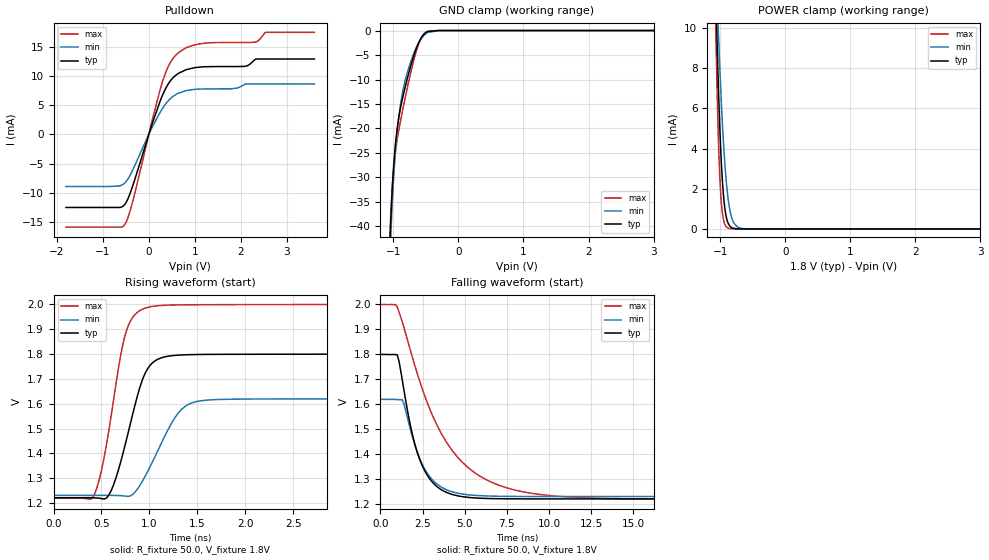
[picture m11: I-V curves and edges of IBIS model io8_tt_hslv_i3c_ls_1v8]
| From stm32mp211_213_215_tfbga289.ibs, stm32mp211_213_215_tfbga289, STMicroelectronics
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[Model]   io8_tt_hslv_i3c_ls_1v8
Model_type I/O_open_drain
Polarity   Non-Inverting
Enable   Active-Low
| CAP_THRESHOLD on pad IOTT is "UDTCAPC" :
| Rising=30.0% of vddiov33m   Falling=70.0% of vddiov33m
| C_comp min and max val. don't necessarily correlate with the min and max pvt
| but are the smallest and greatest pad capacitance found.
| var   typ   min   max
C_comp   1.23170pF  1.11694pF  1.38090pF
|C_comp_pulldown   1.23170pF  1.11694pF  1.38090pF
Vinl = 810.0mV
Vinh = 1.0V
Vmeas = 900.0mV   | Reference voltage for timing measurements
Cref  = 50.0pF   | Timing specification test load capacitance value
Rref  = 1.0MOhm   | Timing specification test load resistance value
Vref  = 990.0mV   | Timing specification test load voltage
[Model Spec]
| TIME_THRESHOLD on pin ZIV08M is "CMOS" :
| Rising=50.0% of vddv08m   Falling=50.0% of vddv08m
Vinl 675.70000mV 623.70000mV 735.70000mV
Vinh 1.12730V 1.01130V 1.24930V
| variable   typ   min   max
[Temperature Range] 25.0 125.0 -40.0
| variable   typ   min   max
[Voltage Range] 1.8V 1.62V 2.0V
| variable   typ   min   max
[POWER Clamp Reference] 1.8V 1.62V 2.0V
| variable   typ   min   max
[GND Clamp Reference] 0V 0V 0V
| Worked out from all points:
|   slope of the pulldown table from 0 to 0.27 V, typ, clamps not added: 43.9 ohm
|   GND clamp passes 1 mA (typ) near -0.55 V on its own axis
|   POWER clamp passes 1 mA (typ) near -0.93 V on its own axis
|   rising waveform, R_fixture 50.0, V_fixture 1.8V: 20-80 % time 236ps typ, 306ps min, 202ps max; typ from 1.22 V to 1.8 V
|   falling waveform, R_fixture 50.0, V_fixture 1.8V: 20-80 % time 1.28ns typ, 1.33ns min, 3.09ns max; typ from 1.8 V to 1.22 V
[POWER Clamp]
-1.8V     152.1mA    105.6mA    221.1mA
-1.07V    12.07mA    13.61mA    10.38mA
-1.05V    9.569mA    11.75mA    7.248mA
-1.03V    7.339mA    9.993mA    4.743mA
-1.01V    5.42mA     8.357mA    2.898mA
-990mV    3.841mA    6.859mA    1.662mA
-970mV    2.609mA    5.513mA    906.4uA
-940mV    1.358mA    3.806mA    344.1uA
-880mV    308.2uA    1.548mA    45.5uA
-790mV    28.46uA    298.8uA    2.106uA
-610mV    211.8nA    7.522uA    9.52nA
3.6V      0A         0A         0A
[GND Clamp]
-1.8V     -1.222A    -1.193A    -1.238A
-1.05V    -42.33mA   -45.55mA   -41.2mA
-1.04V    -38.89mA   -42.1mA    -37.88mA
-1.03V    -35.83mA   -38.98mA   -35.06mA
-1.01V    -30.7mA    -33.54mA   -30.61mA
-970mV    -23.47mA   -25.17mA   -24.97mA
-920mV    -18.06mA   -18.06mA   -20.63mA
-870mV    -14.51mA   -13.44mA   -17.13mA
-780mV    -9.532mA   -8.354mA   -11.38mA
-650mV    -3.743mA   -3.581mA   -4.327mA
-490mV    -324.1uA   -556uA     -259.6uA
3.6V      66.06nA    2.767uA    18.5nA
| variable   typ   min   max
[Pullup Reference] 1.8V 1.62V 2.0V
| variable   typ   min   max
[Pulldown Reference] 0V 0V 0V
[Pulldown]
-1.8V     -12.46mA   -8.882mA   -15.82mA
-520mV    -11.93mA   -8.267mA   -15.35mA
-310mV    -7.858mA   -5.414mA   -10.27mA
280mV     6.351mA    4.22mA     8.544mA
440mV     8.829mA    5.894mA    11.87mA
630mV     10.37mA    7.006mA    13.9mA
1.18V     11.56mA    7.771mA    15.57mA
1.8V      11.61mA    7.801mA    15.71mA
2.09V     11.64mA    8.584mA    15.71mA
2.31V     12.8mA     8.642mA    15.76mA
2.54V     12.89mA    8.642mA    17.45mA
3.6V      12.89mA    8.642mA    17.45mA
[Ramp]
dV/dt_r 347.11996mV/235.79817ps 233.32671mV/305.65505ps 468.11487mV/201.7592ps
dV/dt_f 347.15374mV/1.27575ns 233.36791mV/1.32718ns 468.14304mV/3.08635ns
R_load = 50.0
| Removed startup time: 0s 0s 0s  .
| Removed end time: 6.975ns.
[Rising Waveform]
R_fixture   = 50.0
V_fixture   = 1.8V
V_fixture_min = 1.62V
V_fixture_max = 2.0V
0s        1.221V     1.231V     1.22V
425ps     1.221V     1.231V     1.233V
500ps     1.218V     1.231V     1.332V
575ps     1.231V     1.231V     1.488V
750ps     1.439V     1.228V     1.881V
850ps     1.596V     1.244V     1.96V
975ps     1.737V     1.322V     1.988V
1.3ns     1.796V     1.562V     1.998V
1.55ns    1.799V     1.613V     1.999V
6.975ns   1.8V       1.62V      2V
| Removed startup time: 0s 0s 0s  .
| Removed end time: 199.9ns.
[Falling Waveform]
R_fixture   = 50.0
V_fixture   = 1.8V
V_fixture_min = 1.62V
V_fixture_max = 2.0V
0s        1.8V       1.62V      2V
1ns       1.798V     1.619V     1.99V
1.4ns     1.657V     1.602V     1.907V
2.2ns     1.406V     1.406V     1.721V
2.7ns     1.326V     1.333V     1.621V
3.4ns     1.268V     1.279V     1.511V
4.7ns     1.232V     1.243V     1.38V
6.3ns     1.223V     1.233V     1.298V
11.2ns    1.221V     1.231V     1.229V
199.9ns   1.221V     1.231V     1.22V
